(* 	
	Program Name: 	ACS_READ_AXIS_BITS
	Purpose:		(To be used only by Input Scan Function) Copy Drive Bit Arrays into shadow memory for program access 
*)
PROGRAM ACS_READ_AXIS_BITS
VAR_IN_OUT
	Axis:ACS_DRIVE_TYPE;
END_VAR

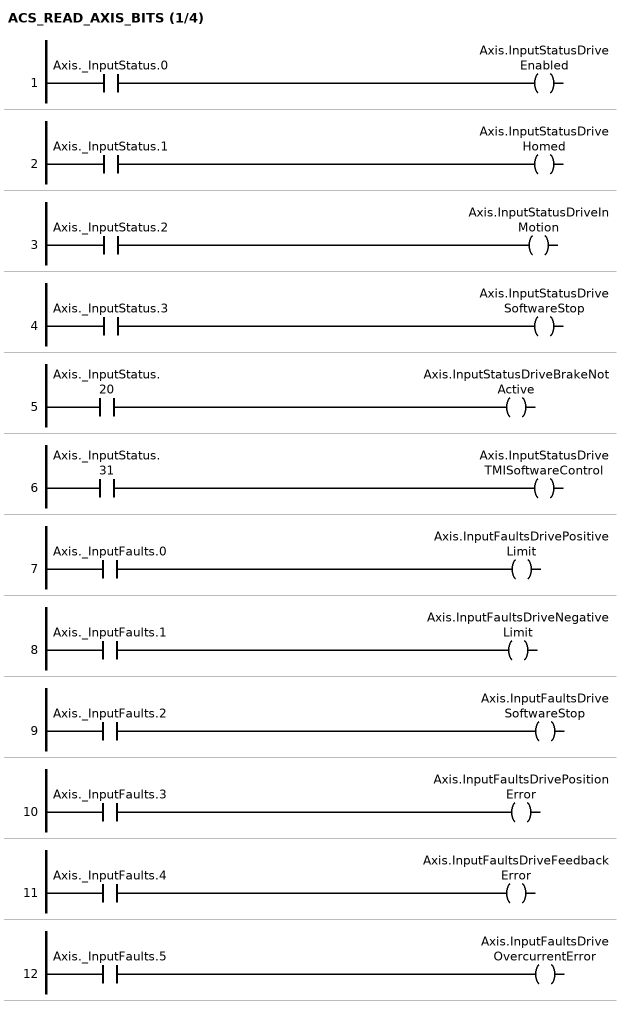
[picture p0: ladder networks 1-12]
// NETWORK 1
Axis.InputStatusDriveEnabled := Axis._InputStatus.0;

// NETWORK 2
Axis.InputStatusDriveHomed := Axis._InputStatus.1;

// NETWORK 3
Axis.InputStatusDriveInMotion := Axis._InputStatus.2;

// NETWORK 4
Axis.InputStatusDriveSoftwareStop := Axis._InputStatus.3;

// NETWORK 5
Axis.InputStatusDriveBrakeNotActive := Axis._InputStatus.20;

// NETWORK 6
Axis.InputStatusDriveTMISoftwareControl := Axis._InputStatus.31;

// NETWORK 7
Axis.InputFaultsDrivePositiveLimit := Axis._InputFaults.0;

// NETWORK 8
Axis.InputFaultsDriveNegativeLimit := Axis._InputFaults.1;

// NETWORK 9
Axis.InputFaultsDriveSoftwareStop := Axis._InputFaults.2;

// NETWORK 10
Axis.InputFaultsDrivePositionError := Axis._InputFaults.3;

// NETWORK 11
Axis.InputFaultsDriveFeedbackError := Axis._InputFaults.4;

// NETWORK 12
Axis.InputFaultsDriveOvercurrentError := Axis._InputFaults.5;

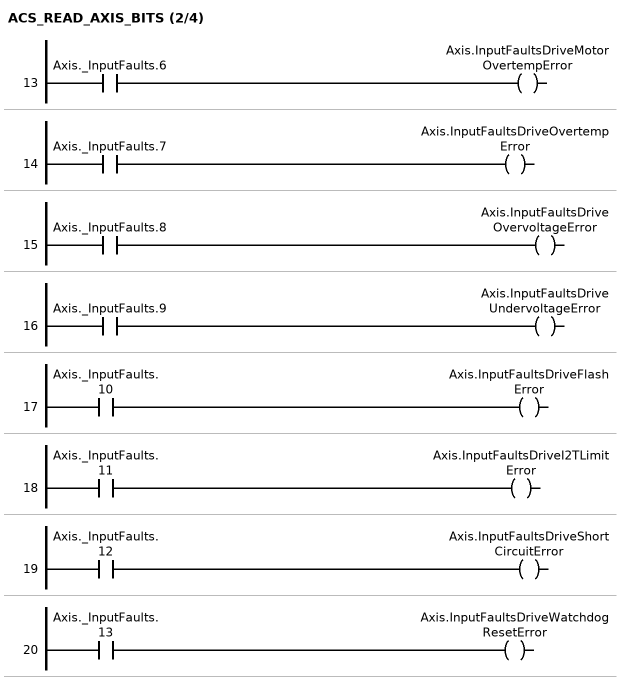
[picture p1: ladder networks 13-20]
// NETWORK 13
Axis.InputFaultsDriveMotorOvertempError := Axis._InputFaults.6;

// NETWORK 14
Axis.InputFaultsDriveOvertempError := Axis._InputFaults.7;

// NETWORK 15
Axis.InputFaultsDriveOvervoltageError := Axis._InputFaults.8;

// NETWORK 16
Axis.InputFaultsDriveUndervoltageError := Axis._InputFaults.9;

// NETWORK 17
Axis.InputFaultsDriveFlashError := Axis._InputFaults.10;

// NETWORK 18
Axis.InputFaultsDriveI2TLimitError := Axis._InputFaults.11;

// NETWORK 19
Axis.InputFaultsDriveShortCircuitError := Axis._InputFaults.12;

// NETWORK 20
Axis.InputFaultsDriveWatchdogResetError := Axis._InputFaults.13;

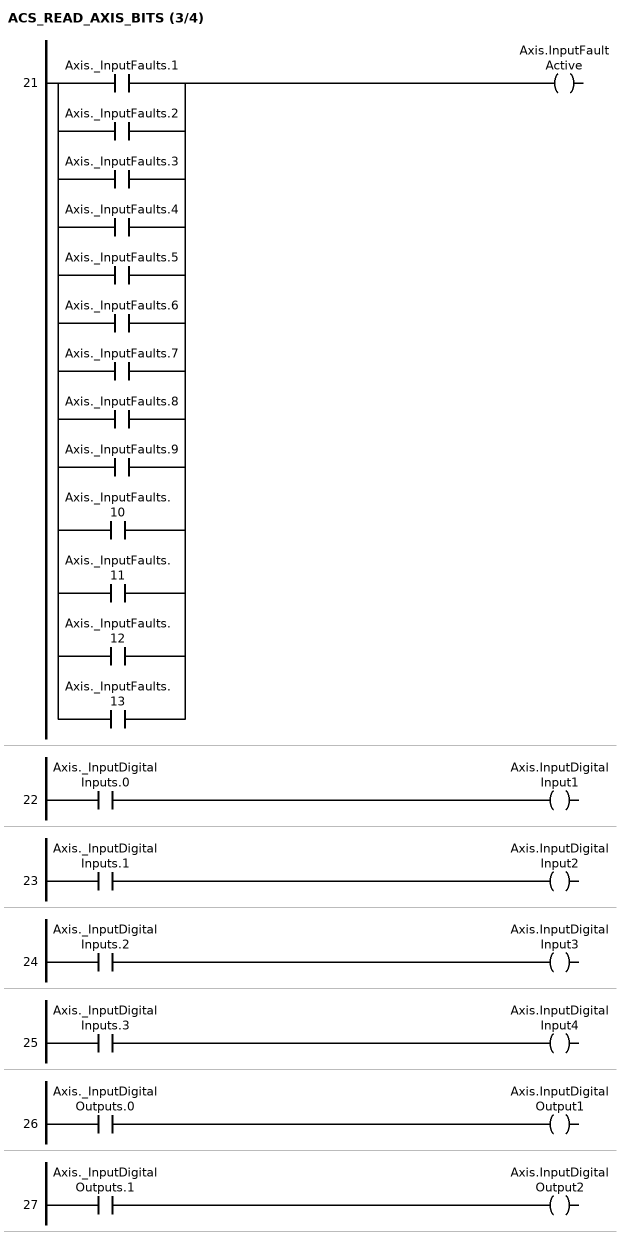
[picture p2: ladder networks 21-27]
// NETWORK 21
Axis.InputFaultActive := Axis._InputFaults.1 OR Axis._InputFaults.2 OR Axis._InputFaults.3 OR Axis._InputFaults.4 OR Axis._InputFaults.5 OR Axis._InputFaults.6 OR Axis._InputFaults.7 OR Axis._InputFaults.8 OR Axis._InputFaults.9 OR Axis._InputFaults.10 OR Axis._InputFaults.11 OR Axis._InputFaults.12 OR Axis._InputFaults.13;

// NETWORK 22
Axis.InputDigitalInput1 := Axis._InputDigitalInputs.0;

// NETWORK 23
Axis.InputDigitalInput2 := Axis._InputDigitalInputs.1;

// NETWORK 24
Axis.InputDigitalInput3 := Axis._InputDigitalInputs.2;

// NETWORK 25
Axis.InputDigitalInput4 := Axis._InputDigitalInputs.3;

// NETWORK 26
Axis.InputDigitalOutput1 := Axis._InputDigitalOutputs.0;

// NETWORK 27
Axis.InputDigitalOutput2 := Axis._InputDigitalOutputs.1;

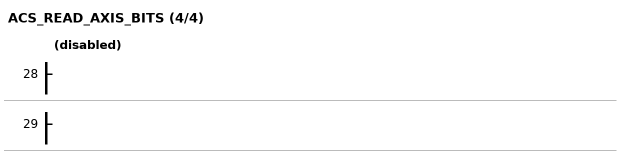
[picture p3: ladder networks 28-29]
// NETWORK 28 (disabled)

// NETWORK 29

END_PROGRAM
